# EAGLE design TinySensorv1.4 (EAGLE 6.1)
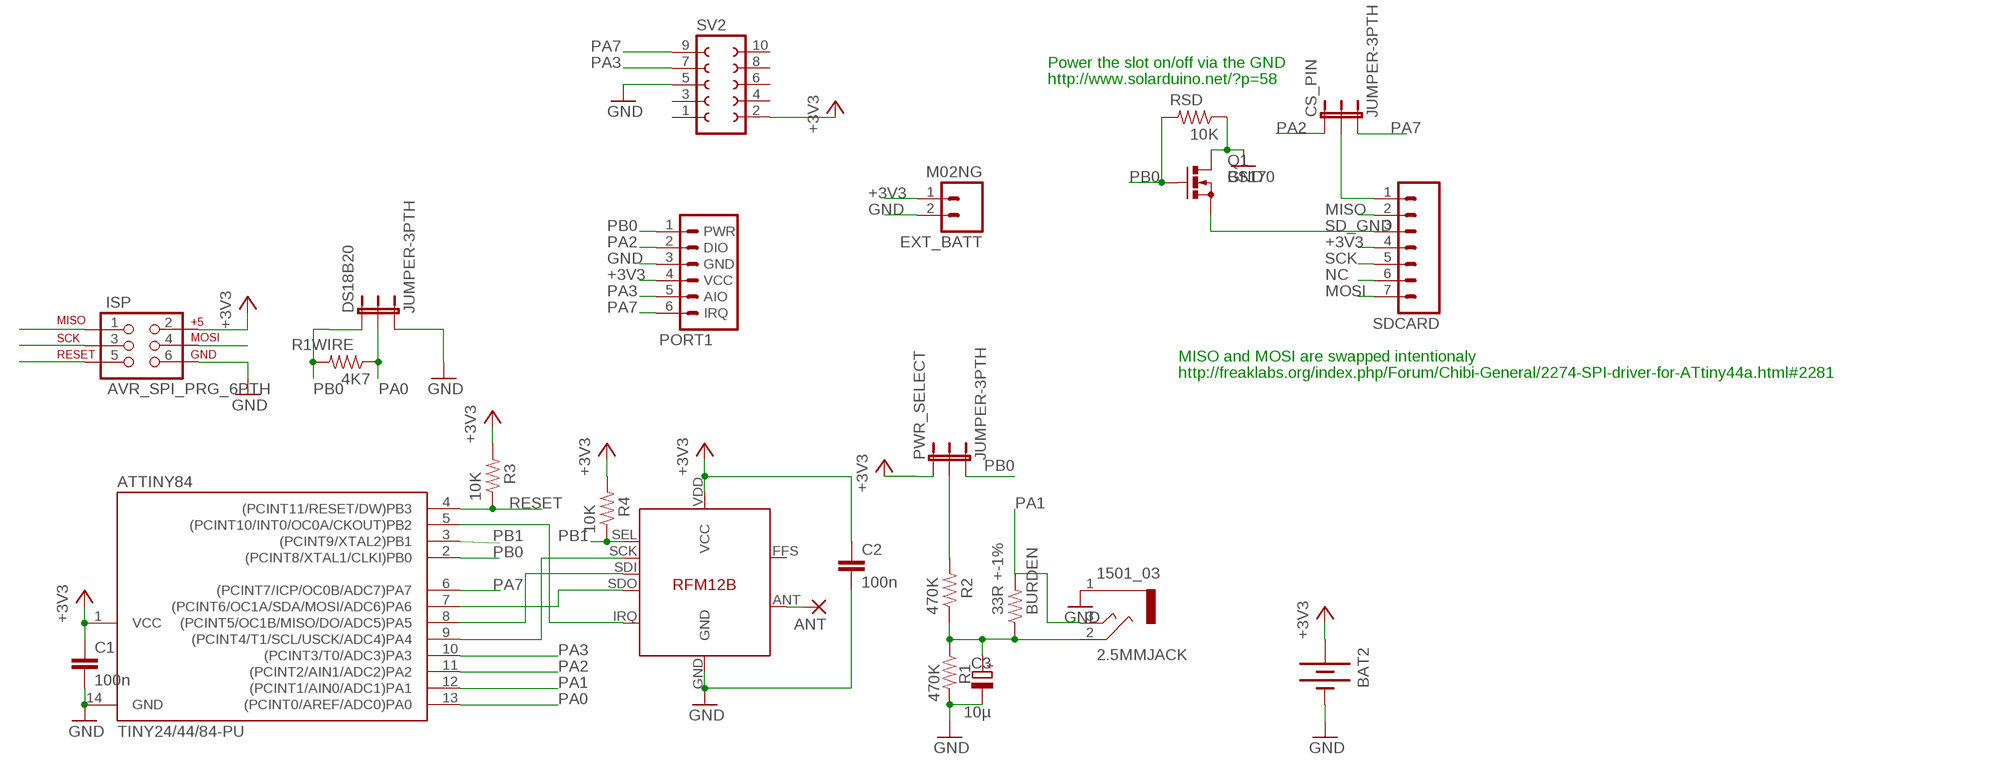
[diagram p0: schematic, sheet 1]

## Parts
2.5MMJACK  1501_03  [1501_03]
ANT  1,6/0,8  [1,6/0,8]
ATTINY84  TINY24/44/84-PU  [DIL14]
BAT2  BATTERY20PTH  [BATTCOM_20MM_PTH]
BURDEN  33R +-1%  RESISTORAXIAL-0.3  [AXIAL-0.3]
C1  100n  C-EU025-024X044  [C025-024X044]
C2  100n  C-EU025-024X044  [C025-024X044]
C3  10µ  CPOL-EUE2.5-6  [E2,5-6]
CS_PIN  JUMPER-3PTH  [1X03]
DS18B20  JUMPER-3PTH  [1X03]
EXT_BATT  M02NG  [1X02]
ISP  AVR_SPI_PRG_6PTH  [2X3]
PORT1  JEEPORT-FEMALE  [1X06_FEMALE_LOCK.010]
PWR_SELECT  JUMPER-3PTH  [1X03]
Q1  BS170  [SOT54E]
R1  470K  RESISTORAXIAL-0.3  [AXIAL-0.3]
R1WIRE  4K7  RESISTORAXIAL-0.3  [AXIAL-0.3]
R2  470K  RESISTORAXIAL-0.3  [AXIAL-0.3]
R3  10K  RESISTORAXIAL-0.3  [AXIAL-0.3]
R4  10K  RESISTORAXIAL-0.3  [AXIAL-0.3]
RFM12B  RFM12B  [RFM12B]
RSD  10K  RESISTORAXIAL-0.3  [AXIAL-0.3]
SDCARD  M07LOCK  [1X07_LOCK]
SV2  FE05-2  [FE05-2]

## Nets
+3V3 [power]: ATTINY84.1(VCC) BAT2.1(+) C1.1 C2.1 EXT_BATT.1 ISP.2 PORT1.4(VCC) PWR_SELECT.1 R3.P$2 R4.P$2 RFM12B.VDD(VCC) SDCARD.4 SV2.2
GND [power]: 2.5MMJACK.1 ATTINY84.14(GND) BAT2.2(-) C1.2 C2.2 C3.- DS18B20.3 EXT_BATT.2 ISP.6 PORT1.3(GND) Q1.D R1.P$2 RFM12B.GND RSD.P$1 SV2.5
MISO: ATTINY84.8((PCINT5/OC1B/MISO/DO/ADC5)PA5) ISP.1 RFM12B.SDI SDCARD.2
MOSI: ATTINY84.7((PCINT6/OC1A/SDA/MOSI/ADC6)PA6) ISP.4 RFM12B.SDO SDCARD.7
N$1: PWR_SELECT.2 R2.P$2
N$3: CS_PIN.2 SDCARD.1
N$6 [power]: ANT.1(P) RFM12B.ANT
N$10: 2.5MMJACK.2 BURDEN.P$1 C3.+ R1.P$1 R2.P$1
NC: SDCARD.6
PA0: ATTINY84.13((PCINT0/AREF/ADC0)PA0) DS18B20.2 R1WIRE.P$1
PA1: 2.5MMJACK.3 ATTINY84.12((PCINT1/AIN0/ADC1)PA1) BURDEN.P$2
PA2: ATTINY84.11((PCINT2/AIN1/ADC2)PA2) CS_PIN.1 PORT1.2(DIO)
PA3: ATTINY84.10((PCINT3/T0/ADC3)PA3) PORT1.5(AIO) SV2.7
PA7: ATTINY84.6((PCINT7/ICP/OC0B/ADC7)PA7) CS_PIN.3 PORT1.6(IRQ) SV2.9
PB0: ATTINY84.2((PCINT8/XTAL1/CLKI)PB0) DS18B20.1 PORT1.1(PWR) PWR_SELECT.3 Q1.G R1WIRE.P$2 RSD.P$2
PB1: ATTINY84.3((PCINT9/XTAL2)PB1) R4.P$1 RFM12B.SEL
PB2: ATTINY84.5((PCINT10/INT0/OC0A/CKOUT)PB2) RFM12B.IRQ
RESET: ATTINY84.4((PCINT11/RESET/DW)PB3) ISP.5 R3.P$1
SCK: ATTINY84.9((PCINT4/T1/SCL/USCK/ADC4)PA4) ISP.3 RFM12B.SCK SDCARD.5
SD_GND: Q1.S SDCARD.3
Unconnected: RFM12B.FFS SV2.1 SV2.3 SV2.4 SV2.6 SV2.8 SV2.10

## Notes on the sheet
- Power the slot on/off via the GND
- http://www.solarduino.net/?p=58
- MISO and MOSI are swapped intentionaly
- http://freaklabs.org/index.php/Forum/Chibi-General/2274-SPI-driver-for-ATtiny44a.html#2281

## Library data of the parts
2.5MMJACK = con-lumberg:1501_03: Klinkensteckverbinder nach JISC 6560, 2,5 mm Jack connectors according to JISC 6560, 2.5 mm Source: http://www.lumberg.com/Produkte/PDFs/1501_03.pdf; OC_FARNELL: 1200127; OC_NEWARK: unknown
ANT = JeeLabs:1,6/0,8: THROUGH-HOLE PAD
ATTINY84 = avr-7:TINY24/44/84
BAT2 = SparkFun:BATTERY: Battery Holders
BURDEN R1 R1WIRE R2-R4 RSD = SparkFun:RESISTOR: Resistor
C1 C2 = rcl:C-EU: CAPACITOR, European symbol
C3 = rcl:CPOL-EU: POLARIZED CAPACITOR, European symbol
CS_PIN DS18B20 PWR_SELECT = SparkFun:JUMPER-3
EXT_BATT = SparkFun:M02NG
ISP = SparkFun:AVR_SPI_PRG_6: AVR ISP 6 Pin This is the reduced ISP connector for AVR programming. Common on Arduino. This footprint will take up less PCB space and can be used with a 10-pin to 6-pin adapter such as SKU: BOB-08508
PORT1 = JeeParts:JEEPORT: PIN HEADER
Q1 = transistor-small-signal:BS170: N-CHANNEL MOS FET
RFM12B = JeeLabs:RFM12B
SDCARD = SparkFun:M07: Header 7 Standard 7-pin 0.1" header. Use with straight break away headers (SKU : PRT-00116), right angle break away headers (PRT-00553), swiss pins (PRT-00743), machine pins (PRT-00117), and female headers (PRT-00115). NOTES ON THE VARIANTS LOCK and LOCK_LONGPADS... This footprint was designed to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
SV2 = con-lsta:FE05-2: FEMALE HEADER; OC_FARNELL: unknown; OC_NEWARK: unknown

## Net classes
0 default: width 0.356 mm, drill 0.356 mm, clearance 0.356 mm
1 power: width 0.406 mm, drill 0.356 mm, clearance 0.406 mm

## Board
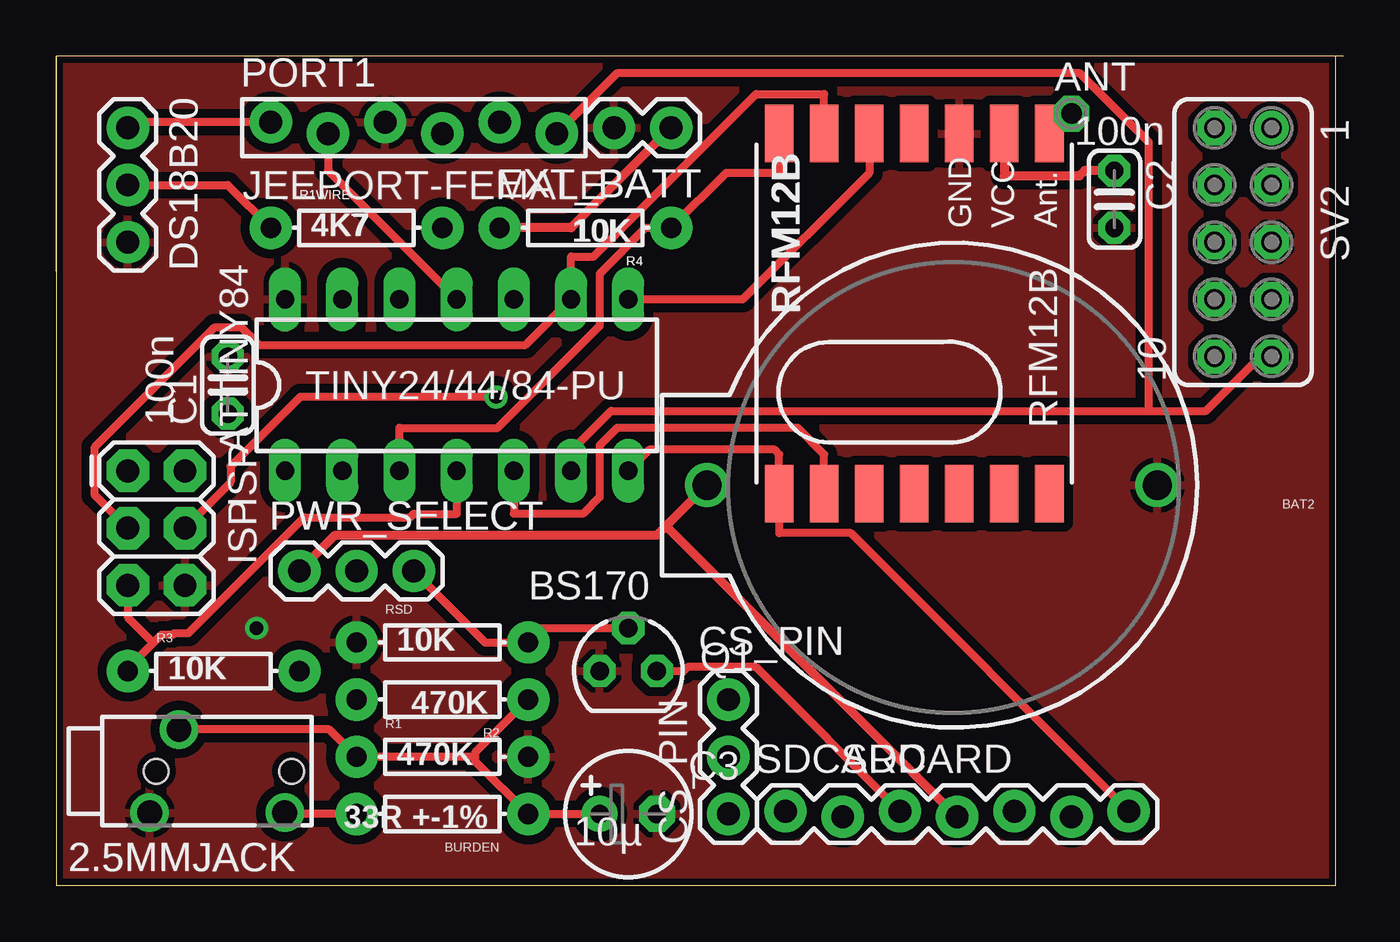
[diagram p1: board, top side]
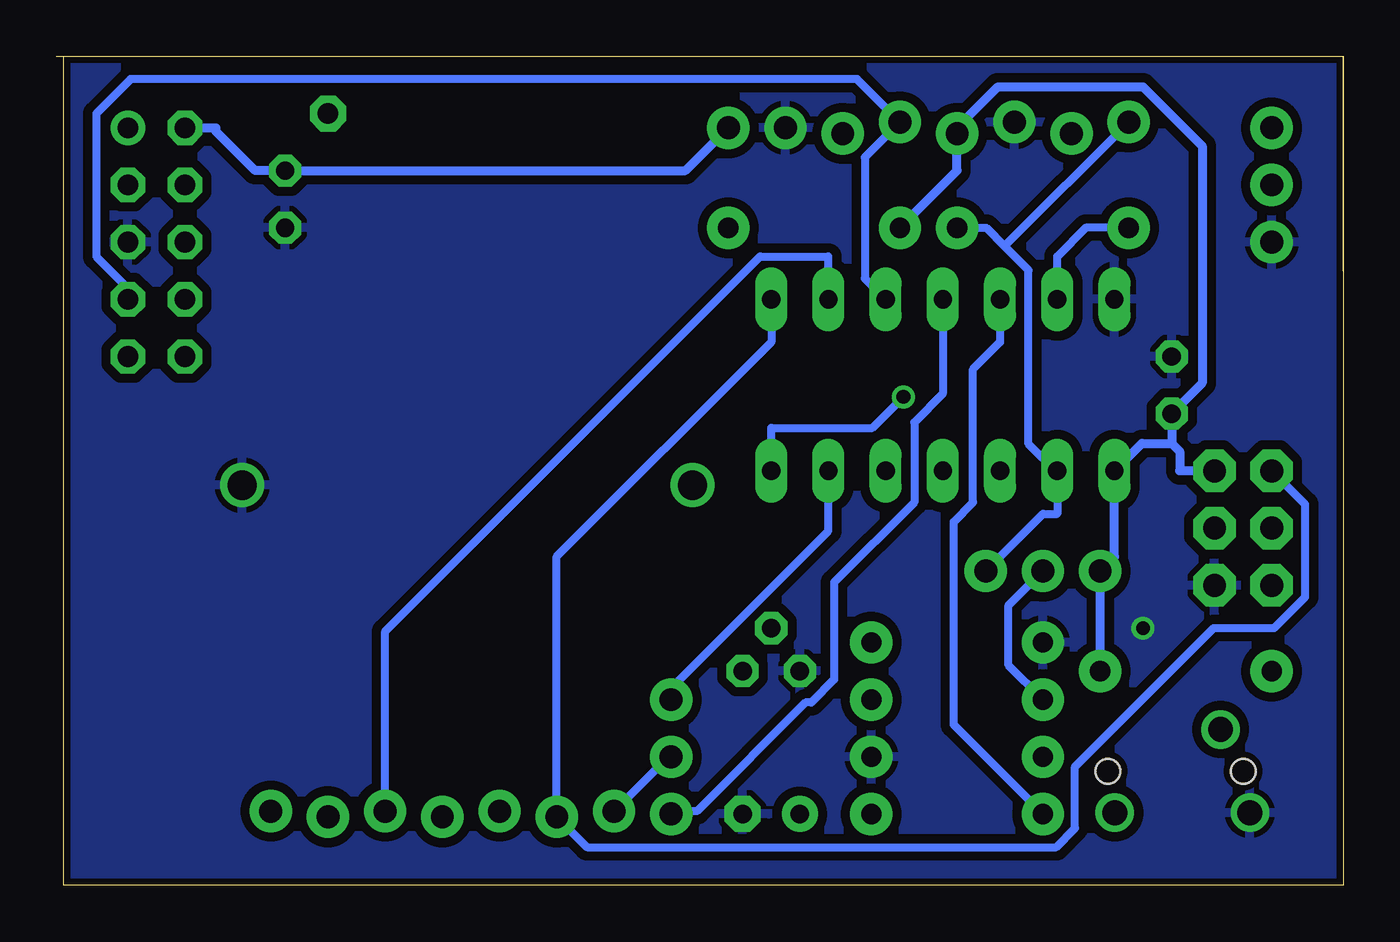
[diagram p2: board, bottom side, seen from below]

Size 57.15 x 36.83 mm. Coordinates in mm from the lower left corner, seen from the top.
Outline: 56.82,36.82 56.82,0 0,0 0,27.3
Outline: 0,27.3 0,36.83
Outline: 0,36.83 0,27.3
Outline: 57.15,36.83 0,36.83
Copper layers (1*16): Top 0.035mm / dielectric 1.5mm / Bottom 0.035mm
Design rules: minimum track width 12mil, minimum drill 24mil, track to track 12mil, track to pad 12mil, pad to pad 12mil, via to via 14mil, smd to smd 10mil, copper to edge 12mil, drill to drill 8mil, minimum pad ring 12mil, minimum via ring 8mil, stop-mask expansion 4mil, vias tented up to drill 0mil, thermal gap 10mil

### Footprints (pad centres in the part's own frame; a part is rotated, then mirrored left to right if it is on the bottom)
1501_03 = drill 1.1 pad 1.7: 1 -1.85,0.3; 2 1.85,-1; 3 -1.85,-5.7 | hole 1.1: 0,0; 0,-6
1,6/0,8 = drill 0.9 pad 1.6 octagon: 1 0,0
DIL14 = drill 0.813 long: 1 -7.62,-3.81; 2 -5.08,-3.81; 3 -2.54,-3.81; 4 0,-3.81; 5 2.54,-3.81; 6 5.08,-3.81; 7 7.62,-3.81; 8 7.62,3.81; 9 5.08,3.81; 10 2.54,3.81; 11 0,3.81; 12 -2.54,3.81; 13 -5.08,3.81; 14 -7.62,3.81
BATTCOM_20MM_PTH = drill 1.3: 1 20,0; 2 0,0
AXIAL-0.3 = drill 0.9 pad 1.88: P$1 -3.81,0; P$2 3.81,0
C025-024X044 = drill 0.813 octagon: 1 -1.27,0; 2 1.27,0
E2,5-6 = drill 0.813 pad 1.6: + -1.27,0 | drill 0.813 pad 1.6 octagon: - 1.27,0
1X03 = drill 1.016 pad 1.88: 1 0,0; 2 2.54,0; 3 5.08,0
1X02 = drill 1.016 pad 1.88: 1 0,0; 2 2.54,0
2X3 = drill 1.016 pad 1.88 octagon: 1 0,0; 2 0,2.54; 3 2.54,0; 4 2.54,2.54; 5 5.08,0; 6 5.08,2.54
1X06_FEMALE_LOCK.010 = drill 1.016 pad 1.88: 1 0,0.254; 2 2.54,-0.254; 3 5.08,0.254; 4 7.62,-0.254; 5 10.16,0.254; 6 12.7,-0.254
SOT54E = drill 0.813 octagon: D -1.27,0; G 0,1.905; S 1.27,0
RFM12B = smd 2.54 x 1.27: ANT 8,-6; FFS -8,2; GND 8,-2; IRQ -8,4; P$8 -8,0; P$9 -8,-2; P$10 -8,-4; P$12 -8,-6; P$16 8,0; SCK 8,4; SDI 8,2; SDO -8,6; SEL 8,6; VDD 8,-4
1X07_LOCK = drill 1.016 pad 1.88: 1 0,0.127; 2 2.54,-0.127; 3 5.08,0.127; 4 7.62,-0.127; 5 10.16,0.127; 6 12.7,-0.127; 7 15.24,0.127
FE05-2 = drill 0.914: 1 -5.08,1.27 | drill 0.914 octagon: 2 -5.08,-1.27; 3 -2.54,1.27; 4 -2.54,-1.27; 5 0,1.27; 6 0,-1.27; 7 2.54,1.27; 8 2.54,-1.27; 9 5.08,1.27; 10 5.08,-1.27

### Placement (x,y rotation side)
2.5MMJACK  4.45,5.08 90 top
ANT  45.09,34.29 0 top
ATTINY84  17.78,22.23 0 top
BAT2  48.9,17.78 180 top
BURDEN  17.14,3.17 180 top
C1  7.62,22.23 90 top
C2  46.99,30.48 270 top
C3  25.4,3.17 0 top
CS_PIN  29.84,3.17 90 top
DS18B20  3.17,33.66 270 top
EXT_BATT  27.3,33.66 180 top
ISP  3.17,18.41 270 top
PORT1  9.53,33.66 0 top
PWR_SELECT  10.79,13.97 0 top
Q1  25.4,9.53 0 top
R1  17.14,5.71 0 top
R1WIRE  13.34,29.21 0 top
R2  17.14,8.26 180 top
R3  6.99,9.53 0 top
R4  23.5,29.21 180 top
RFM12B  38.1,25.4 90 top
RSD  17.14,10.79 0 top
SDCARD  32.38,3.17 0 top
SV2  52.7,28.57 270 top

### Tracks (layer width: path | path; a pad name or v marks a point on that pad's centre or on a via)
+3V3
  Top 0.406: EXT_BATT.1 22.86,29.21 R4.P$2 | 27.08,15.97 BAT2.1 | PWR_SELECT.1 12.39,15.56 26.68,15.56 27.08,15.97 | SDCARD.4 27.08,15.97 | C2.1 45.67,31.75 45.44,31.52 42.1,31.52 RFM12B.VDD
  Bottom 0.406: ISP.2 7.26,18.41 7.26,19.28 7.62,19.63 | 7.62,19.63 8.94,19.63 ATTINY84.1 10.16,14.61 PWR_SELECT.1 R3.P$2 | R4.P$2 17.14,31.75 PORT1.4 17.14,33.66 15.33,35.47 8.89,35.47 6.26,32.84 6.26,22.32 C1.1 7.62,19.63 | SV2.2 50.06,33.66 50.06,33.5 48.31,31.75 C2.1 29.21,31.75 EXT_BATT.1
GND  (via drill 0.61 pad 1.02)
  other vias: 8.89,11.43
  pour Bottom: -1.27,38.1 58.42,38.1 58.42,-1.27 -1.27,-1.27
  pour Top: -2.54,39.37 60.96,39.37 60.96,-2.54 -2.54,-2.54
MISO
  Top 0.356: RFM12B.SDI 36.1,31.65 30.49,26.04 ATTINY84.8
  Bottom 0.356: ISP.1 1.69,16.93 1.69,12.81 3.07,11.43 5.75,11.43 11.91,5.27 11.91,2.54 12.75,1.71 33.58,1.71 SDCARD.2 34.92,14.61 25.4,24.13 ATTINY84.8
MOSI  (via drill 0.61 pad 1.02)
  Top 0.356: v19.53,21.7 10.83,21.7 7.74,18.62 7.74,17.9 ISP.4 | SDCARD.7 35.28,15.65 32.1,15.65 RFM12B.SDO 32.1,19.15 31.87,19.39 26.37,19.39 ATTINY84.7
  Bottom 0.356: ATTINY84.7 25.4,20.32 20.91,20.32 v19.53,21.7
N$1
  Bottom 0.356: R2.P$2 14.86,9.78 14.86,12.45 PWR_SELECT.2
N$3
  Bottom 0.356: SDCARD.1 29.97,5.71 CS_PIN.2
N$6
  Top 0.406: 44.2,33.4 RFM12B.ANT 44.2,33.53 44.96,34.29 ANT.1
N$10
  Top 0.356: C3.+ BURDEN.P$1 18.61,5.52 18.61,5.71 | R2.P$1 18.61,5.91 18.61,5.71 | 18.61,5.71 R1.P$1 12.12,6.93 2.5MMJACK.2
PA0
  Top 0.356: DS18B20.2 7.62,31.11 R1WIRE.P$1
  Bottom 0.356: ATTINY84.13 12.7,27.94 11.43,29.21 R1WIRE.P$1
PA1
  Top 0.356: BURDEN.P$2 10.2,3.17 2.5MMJACK.3
  Bottom 0.356: ATTINY84.12 15.24,24.13 16.43,22.94 16.43,17.02 17.3,16.15 17.3,7.14 BURDEN.P$2
PA2
  Top 0.356: PORT1.2 12.06,31.75 ATTINY84.11
  Bottom 0.356: CS_PIN.1 29.72,3.3 28.7,3.3 23.88,8.13 23.62,8.13 22.61,9.14 22.61,13.46 19.05,17.02 19.05,20.57 17.78,21.84 17.78,25.91 ATTINY84.11
PA3
  Bottom 0.356: ATTINY84.10 21.25,26.96 21.25,32.35 PORT1.5 19.81,34.04 21.59,35.81 53.85,35.81 55.37,34.29 55.37,27.94 54.1,26.67 54.1,26.16 SV2.7
PA7
  Top 0.356: 48.51,21.08 24.64,21.08 22.86,19.3 22.86,18.54 ATTINY84.6 | 48.51,21.08 51.05,21.08 53.34,23.37 53.85,23.37 SV2.9 | 48.51,21.08 48.51,33.02 45.47,36.07 24.89,36.07 22.35,33.53 PORT1.6
  Bottom 0.356: ATTINY84.6 22.86,18.29 22.86,15.75 29.72,8.89 29.72,8.38 CS_PIN.3
PB0
  Top 0.356: PORT1.1 3.43,33.91 DS18B20.1 | PWR_SELECT.3 19.05,10.79 RSD.P$2 21.59,11.43 Q1.G
  Bottom 0.356: 15.04,28.4 PORT1.1 | R1WIRE.P$2 15.85,29.21 15.04,28.4 | 12.7,18.34 13.97,19.61 13.97,27.33 15.04,28.4 | 12.7,18.34 12.7,18.27 12.7,17.46 12.7,16.51 13.34,16.51 PWR_SELECT.3 | ATTINY84.2 12.7,18.34
PB1
  Top 0.356: ATTINY84.3 15.24,20.32 19.59,20.32 24.14,24.87 24.14,27.18 26.17,29.21 R4.P$1 29.74,31.65 32.1,31.65 RFM12B.SEL
PB2
  Top 0.356: ATTINY84.5 20.32,16.51 23.39,16.51 24.13,17.25 24.13,19.55 24.9,20.32 32.93,20.32 34.1,19.15 RFM12B.IRQ
RESET
  Top 0.356: ATTINY84.4 17.78,16.51 15.88,16.51 15.71,16.35 11.02,16.35 5.88,11.21 5.24,11.21 5.18,11.14 4.67,11.14 4.31,10.78 | R3.P$1 3.71,10.06 3.71,10.18 4.31,10.78 | 4.31,10.78 3.17,11.91 ISP.5
SCK
  Top 0.356: ISP.3 1.71,17.34 1.71,19.46 7.04,24.8 8.21,24.8 9,24 20.83,24 ATTINY84.9 22.86,27.94 23.87,27.94 31.08,35.15 34.1,35.15 RFM12B.SCK
  Bottom 0.356: ATTINY84.9 22.86,27.94 25.89,27.94 42.55,11.29 SDCARD.5
SD_GND
  Top 0.356: Q1.S 27.86,9.53 28.04,9.7 31.06,9.7 SDCARD.3

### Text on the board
_tsilk: DS18B20 | PORT1 | 100n | EXT_BATT | JEEPORT-FEMALE | R1WIRE | 10K | 4K7 | GND | VCC | Ant. | R4 | RFM12B | TINY24/44/84-PU | 100n | RFM12B | ISP | PWR_SELECT | BS170 | CS_PIN | 10K | 10K | SDCARD | 2.5MMJACK | 10µ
